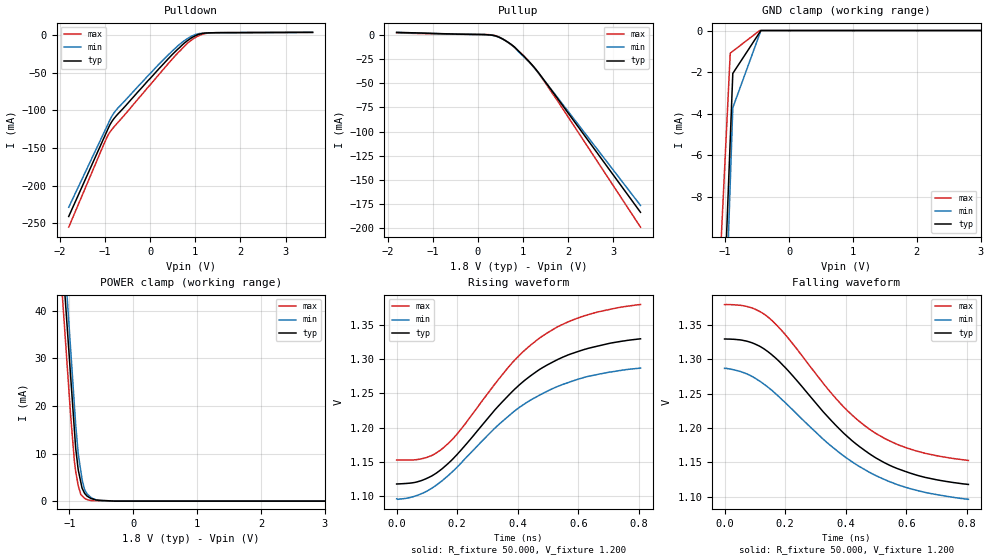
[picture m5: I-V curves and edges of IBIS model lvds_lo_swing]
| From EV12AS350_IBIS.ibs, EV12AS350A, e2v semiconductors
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[Model]   lvds_lo_swing
Model_type Output
Vref=1.200E+00
Rref=5.000E+01
Cref=5.000E-12
Vmeas=1.200E+00
C_comp   8.430E-13   7.910E-13   8.950E-13
[Voltage Range]   1.800E+00   1.700E+00   1.900E+00
[POWER Clamp Reference]   1.800E+00   1.700E+00   1.900E+00
[GND Clamp Reference]   0.000E+00   0.000E+00   0.000E+00
[Pullup Reference]   1.800E+00   1.700E+00   1.900E+00
[Pulldown Reference]   0.000E+00   0.000E+00   0.000E+00
[Temperature Range]   25   110   -40
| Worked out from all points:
|   slope of the pulldown table from 0 to 0.27 V, typ, clamps not added: 15.2 ohm
|   slope of the pullup table from 0 to 0.27 V, typ, clamps not added: 499 ohm
|   POWER clamp passes 1 mA (typ) near -0.72 V on its own axis
|   rising waveform, R_fixture 50.000, V_fixture 1.200: 20-80 % time 282ps typ, 297ps min, 270ps max; typ from 1.12 V to 1.33 V
|   falling waveform, R_fixture 50.000, V_fixture 1.200: 20-80 % time 284ps typ, 312ps min, 275ps max; typ from 1.33 V to 1.12 V
[GND Clamp]
-1.9V     -83.54mA   -96.4mA    -63.1mA
-1.8V     -75.55mA   -87.32mA   -56.77mA
-1.7V     -67.56mA   -78.23mA   -50.45mA
-920mV    -5.262mA   -7.352mA   -1.091mA
-880mV    -2.067mA   -3.717mA   -996.3uA
-460mV    -93.95uA   -169uA     0A
-440mV    0A         0A         0A
0V        0A         0A         0A
3.4V      0A         0A         0A
3.6V      0A         0A         0A
3.8V      0A         0A         0A
[POWER Clamp]
-2V       222.1mA    236.6mA    216.1mA
-1.6V     145.3mA    156.4mA    138.5mA
-1.04V    37.95mA    44.12mA    29.87mA
-980mV    26.45mA    32.1mA     18.23mA
-920mV    14.94mA    20.07mA    8.355mA
-900mV    11.11mA    16.06mA    6.238mA
-860mV    6.551mA    9.912mA    3.219mA
-800mV    2.726mA    4.553mA    1.138mA
-760mV    1.624mA    2.385mA    581.8uA
-640mV    474.4uA    593.9uA    104.1uA
-460mV    137.9uA    47.59uA    43.66uA
3.7V      0A         0A         0A
[Pullup]
-1.8V     2.5mA      2.273mA    1.809mA
300mV     -406.8uA   -485uA     -168.8uA
400mV     -1.378mA   -1.516mA   -1.115mA
540mV     -4.19mA    -4.312mA   -4.09mA
800mV     -12.28mA   -12.74mA   -12.58mA
1.12V     -27.13mA   -27.54mA   -27.16mA
1.36V     -40.35mA   -40.65mA   -40.88mA
1.76V     -65.71mA   -64.75mA   -68.08mA
3.6V      -183.5mA   -176.4mA   -198.8mA
[Pulldown]
-1.8V     -240.9mA   -228.6mA   -255.1mA
-1.02V    -136.5mA   -129.6mA   -144.5mA
-900mV    -120.6mA   -114.3mA   -130mA
-820mV    -112.6mA   -105.3mA   -123.5mA
-720mV    -105.3mA   -97.44mA   -116.6mA
160mV     -47.12mA   -40.99mA   -54.92mA
620mV     -18.47mA   -14.01mA   -23.5mA
880mV     -5.168mA   -2.725mA   -8.34mA
1.1V      1.369mA    2.123mA    -236.9uA
1.34V     3.095mA    3.061mA    2.958mA
3.6V      3.646mA    3.707mA    3.687mA
[Rising Waveform]
R_fixture = 50.000
V_fixture = 1.200
V_fixture_min = 1.200
V_fixture_max = 1.200
|  time   V(typ)   V(min)   V(max)
0s        1.118V     1.096V     1.153V
90ps      1.124V     1.105V     1.155V
150ps     1.14V      1.122V     1.169V
210ps     1.166V     1.147V     1.196V
325ps     1.226V     1.2V       1.264V
385ps     1.254V     1.223V     1.296V
490ps     1.29V      1.252V     1.336V
545ps     1.302V     1.262V     1.35V
625ps     1.315V     1.274V     1.364V
805ps     1.33V      1.287V     1.38V
[Falling Waveform]
R_fixture = 50.000
V_fixture = 1.200
V_fixture_min = 1.200
V_fixture_max = 1.200
|  time   V(typ)   V(min)   V(max)
0s        1.33V      1.287V     1.38V
80ps      1.326V     1.278V     1.376V
145ps     1.311V     1.259V     1.361V
205ps     1.286V     1.235V     1.334V
380ps     1.198V     1.164V     1.237V
430ps     1.178V     1.148V     1.215V
490ps     1.159V     1.133V     1.195V
555ps     1.144V     1.12V      1.179V
630ps     1.132V     1.109V     1.167V
805ps     1.118V     1.096V     1.153V
[Ramp]
dV/dt_r   1.2720E-01/2.8240E-10   1.1454E-01/2.9690E-10   1.3626E-01/2.7300E-10
dV/dt_f   1.2720E-01/2.8430E-10   1.1454E-01/3.1159E-10   1.3626E-01/2.7525E-10
R_load = 50
